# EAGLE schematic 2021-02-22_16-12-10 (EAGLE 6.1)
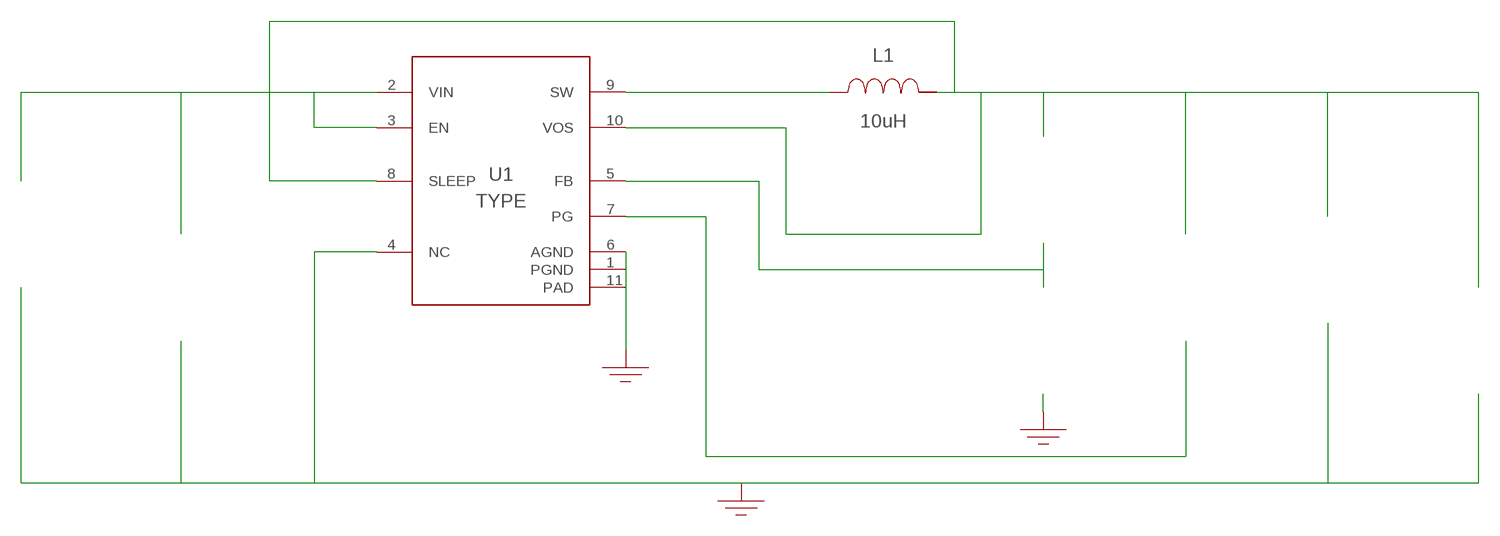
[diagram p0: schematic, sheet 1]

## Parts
CIN  2.2uF  GRM21BR71E225KA73LGRM21BR71E225KA73L  [0805]  (not placed on a sheet)
COUT  22uF  C1608X5R1A226M080ACC1608X5R1A226M080AC  [0603]  (not placed on a sheet)
GND8  WB_GND  WB_GNDWB_GND  [WB_GND]
GND9  WB_GND  WB_GNDWB_GND  [WB_GND]
GND11  WB_GND  WB_GNDWB_GND  [WB_GND]
IOUT  WB_CURRENT_LOAD  WB_CURRENT_LOADWB_CURRENT_LOAD  [WB_CURRENT_LOAD]  (not placed on a sheet)
L1  10uH  NPI54C100MTRFNPI54C100MTRF  [IND_NPI54C]
RFBB  383k  CRCW0402383KFKEDCRCW0402383KFKED  [0402]  (not placed on a sheet)
RFBT  2M  CRCW04022M00FKEDCRCW04022M00FKED  [0402]  (not placed on a sheet)
RPG  100k  CRCW0402100KFKEDCRCW0402100KFKED  [0402]  (not placed on a sheet)
U1  TPS62175DQCR  TPS62175DQCRTPS62175DQCR  [DQC0010A]
VIN  WB_BATTERY  WB_BATTERYWB_BATTERY  [WB_BATTERY]  (not placed on a sheet)

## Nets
0: Cin.2@2 Cout.2@2 GND8.1 GND9.1 GND11.1 Iout.-@2 Rfbb.1@1 U1.1(PGND) U1.4(NC) U1.6(AGND) Vin.-@2
1: Rpg.2@2 U1.7(PG)
2: Cout.1@1 Iout.+@1 L1.2 Rfbt.1@1 Rpg.1@1 U1.8(SLEEP) U1.10(VOS)
3: L1.1 U1.9(SW)
4: Rfbb.2@2 Rfbt.2@2 U1.5(FB)
5: Cin.1@1 U1.2(VIN) U1.3(EN) Vin.+@1
Unconnected: CIN.1 CIN.2 COUT.1 COUT.2 IOUT.1(+) IOUT.2(-) RFBB.1 RFBB.2 RFBT.1 RFBT.2 RPG.1 RPG.2 VIN.1(+) VIN.2(-)

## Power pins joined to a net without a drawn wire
PAD: U1.11(PAD)

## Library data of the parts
CIN = AcceleratedDesigns_Lib:GRM21BR71E225KA73L; Cap: 2.2E-6; ESR: 0.0050; IRMS: 0.0; Manufacturer_Name: MuRata; Manufacturer_Part_Number: GRM21BR71E225KA73L; VDC: 25.0; Vendor: MuRata
COUT = AcceleratedDesigns_Lib:C1608X5R1A226M080AC; Cap: 2.2E-5; Datasheet_URL: https://product.tdk.com/en/search/capacitor/ceramic/mlcc/info?part%5Fno%3DC1608X5R1A226M080AC; ESR: 0.00371; IRMS: 2.69936; Manufacturer_Name: TDK; Manufacturer_Part_Number: C1608X5R1A226M080AC; VDC: 10.0; Vendor: TDK
GND8 GND9 GND11 = AcceleratedDesigns_Lib:WB_GND; Manufacturer_Name: WB_GND; Manufacturer_Part_Number: WB_GND; PowerPortType: POWER_GROUND; Value: Value
IOUT = AcceleratedDesigns_Lib:WB_CURRENT_LOAD; Manufacturer_Name: WB_CURRENT_LOAD; Manufacturer_Part_Number: WB_CURRENT_LOAD; PowerPortType: POWER_GROUND; Value: Value
L1 = AcceleratedDesigns_Lib:NPI54C100MTRF; DCR: 0.09; IDC: 1.8; L: 1.0E-5; Manufacturer_Name: NIC Components; Manufacturer_Part_Number: NPI54C100MTRF; Vendor: NIC Components
RFBB = AcceleratedDesigns_Lib:CRCW0402383KFKED; Manufacturer_Name: Vishay-Dale; Manufacturer_Part_Number: CRCW0402383KFKED; Power: 0.063; Resistance: 383000.0; Tolerance: 1.0; Vendor: Vishay-Dale
RFBT = AcceleratedDesigns_Lib:CRCW04022M00FKED; Manufacturer_Name: Vishay-Dale; Manufacturer_Part_Number: CRCW04022M00FKED; Power: 0.063; Resistance: 2000000.0; Tolerance: 1.0; Vendor: Vishay-Dale
RPG = AcceleratedDesigns_Lib:CRCW0402100KFKED; Manufacturer_Name: Vishay-Dale; Manufacturer_Part_Number: CRCW0402100KFKED; Power: 0.063; Resistance: 100000.0; Tolerance: 1.0; Vendor: Vishay-Dale
U1 = AcceleratedDesigns_Lib:TPS62175DQCR; Manufacturer: Texas Instruments; Manufacturer_Name: Texas Instruments; Manufacturer_Part_Number: TPS62175DQCR; PartNumber: TPS62175DQCR; RefDes: RefDes; TYPE: TYPE; Value: Value
VIN = AcceleratedDesigns_Lib:WB_BATTERY; Manufacturer_Name: WB_BATTERY; Manufacturer_Part_Number: WB_BATTERY; PowerPortType: POWER_GROUND; Value: Value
